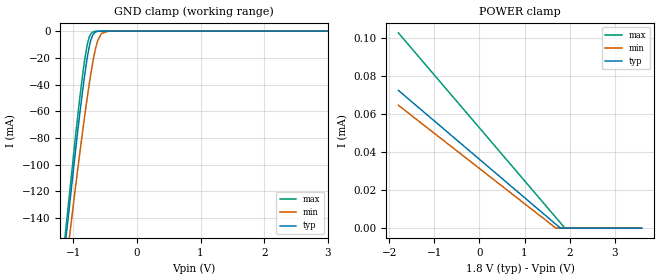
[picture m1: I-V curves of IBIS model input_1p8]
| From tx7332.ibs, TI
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|   input_1p8 Model
[Model]   input_1p8
Model_type   Input
Vinl = 0.45
Vinh = 1.35
|   typ   min   max
C_comp   6.481pF   6.451pF   6.572pF
[Model spec]
|subparameter
Vinl   0.45   0.425   0.475
Vinh   1.35   1.275   1.425
| Where Nom  PVT is Nominal Process, 1.8V, 27C
|   Fast PVT is Strong Process,  1.9V, 0C
|   Slow PVT is Weak Process,   1.7V, 100C
[Voltage Range]   1.8   1.7   1.9
|Junction Temperature
[Temperature Range]   27   100   0
[Power Clamp Reference]   1.8   1.7   1.9
[GND Clamp Reference]   0   0   0
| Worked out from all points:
|   GND clamp passes 1 mA (typ) near -0.66 V on its own axis
[GND Clamp]
|   Voltage   I(typ)   I(min)   I(max)
-1.8V     -470.8mA   -456.6mA   -480.7mA
-1.136V   -164.5mA   -184.2mA   -157.4mA
-957.6mV  -86.91mA   -114.5mA   -75.97mA
-892.8mV  -60.4mA    -90.05mA   -48.62mA
-828mV    -35.92mA   -66.54mA   -24.35mA
-784.8mV  -21.66mA   -51.63mA   -11.65mA
-752.4mV  -12.83mA   -41.01mA   -5.25mA
-693mV    -3.018mA   -23.49mA   -728.7uA
-612mV    -196.9uA   -6.726mA   -57.49uA
-552.6mV  -31.8uA    -1.641mA   -21.26uA
-444.6mV  -9.254uA   -80.57uA   -12.44uA
3.6V      0A         0A         0A
[POWER Clamp]
|   Voltage   I(typ)   I(min)   I(max)
-1.8V     72.28uA    64.48uA    102.4uA
1.694V    2.087uA    64.87nA    5.665uA
1.796V    25.01nA    0A         2.823uA
1.894V    0A         0A         130.7nA
3.6V      0A         0A         0A
